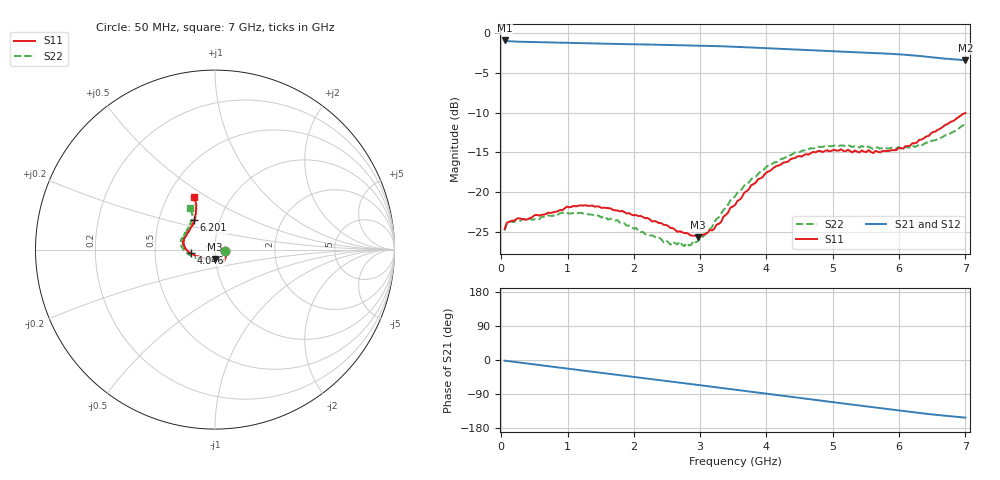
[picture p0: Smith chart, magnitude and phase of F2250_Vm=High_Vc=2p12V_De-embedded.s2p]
! Integrated Device Technology
! Corporate Headquarters
! 6024 Silver Creek Valley Road
! San Jose, CA 95138  USA
! Phone:  1-408-284-8200
! Toll Free:  1-800-223-1366
! Webpage:  http://www.idt.com/
! Timing and RF Division
! 515 Groton Road, Suite 102
! Westford, MA 01886-6024
! Device:  F2250
! Description: Voltage Variable RF Attenuator
! Frequency:  50.0 -  6000.00 MHz
! Package:  3x3 mm Thin QFN Plastic Package: 16 pin
! Ports:  2 RF, 3 DC
!  Pin  1  = GND
!  Pin  2  = NC
!  Pin  3  = RF1  = Port 1
!  Pin  4  = NC
!  Pin  5  = GND
!  Pin  6  = GND
!  Pin  7  = GND
!  Pin  8  = GND
!  Pin  9  = NC
!  Pin 10  = RF2  = Port 2
!  Pin 11  = NC
!  Pin 12  = GND
!  Pin 13  = GND
!  Pin 14  = VCNTRL
!  Pin 15  = VDD
!  Pin 16  = VMODE
! Vcntrl:  2.120 Volts
! Vmode:  +3.300 Volts
! Vdd:  +3.30  Volts
! Current:  1.316 mA
! Data:  The device was measured on a the F2250 evaluation board which has
!  individual transmission lines to the RF pins.  Data was collected
!  using a calibrated network analyzer.  The evaluation board was
!  de-embedded using a TRL calibration technique.
!  The reference plane is the edge of the package pin.
! Misc:  SN 10
!  Action Tracker AT0258
! Date Measured:  2014-11-26
! Date:  2015-10-15  MJV
! Note:
!  Integrated Device Technology supplies this data as a sample of measured
!  data at the package pin for this product.  Your particular data for this
!  product may vary.
!  Data was taken at 25 degrees C.
!  Integrated Device Technology reserves the right to change this data at anytime.
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# GHz S dB R 50
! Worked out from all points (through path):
!   201 points, 50 MHz to 7 GHz, reference 50 ohm
!   highest |S21| = -0.96 dB at 50 MHz (marker M1); lowest = -3.4 dB at 7 GHz (marker M2)
!   group delay of S21, straight-line fit = 61.1 ps
!   lowest |S11| = -25.6 dB at 2.969 GHz (marker M3), VSWR 1.11, Z = 49.6 - j5.19 ohm
!   |S11| at or under -10 dB: start of sweep to end of sweep
!   |S22| runs from -26.8 to -11.5 dB; largest |S21 - S12| = 0.0019
!   S11 on the Smith chart (normalised r, x): 50 MHz: 1.12, -0.02; 4.046 GHz: 0.76, -0.03; 6.201 GHz: 0.75, +0.26; 7 GHz: 0.68, +0.44
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0.05  -24.60 -9.5  -0.96 -1.8  -0.95 -1.8  -24.80 -10.0
0.08475  -23.83 -8.6  -1.03 -2.5  -1.02 -2.5  -23.89 -8.9
0.1195  -23.72 -9.3  -1.06 -3.3  -1.05 -3.2  -23.71 -8.3
0.91875  -22.27 -46.8  -1.24 -21.0  -1.24 -21.1  -22.56 -49.1
1.2315  -21.69 -54.6  -1.31 -27.9  -1.31 -27.9  -22.67 -59.5
1.75275  -22.29 -61.5  -1.40 -39.1  -1.40 -39.1  -23.49 -66.7
2.37825  -23.88 -61.7  -1.49 -52.8  -1.50 -52.8  -25.70 -68.5
2.552  -24.48 -66.1  -1.52 -56.6  -1.52 -56.6  -26.58 -75.0
2.691  -24.90 -73.4  -1.54 -59.7  -1.54 -59.7  -26.19 -82.3
2.7605  -25.14 -75.3  -1.56 -61.3  -1.56 -61.3  -26.77 -86.6
2.969  -25.64 -91.7  -1.59 -66.0  -1.59 -66.0  -26.13 -104.5
3.21225  -24.58 -121.1  -1.65 -71.4  -1.65 -71.5  -23.73 -128.6
3.525  -21.62 -147.8  -1.75 -78.5  -1.75 -78.5  -20.52 -147.2
3.76825  -19.13 -161.2  -1.84 -84.0  -1.84 -84.0  -18.38 -158.4
4.04625  -17.35 -171.2  -1.95 -90.2  -1.95 -90.2  -16.70 -168.9
4.4285  -15.72 178.2  -2.10 -98.6  -2.10 -98.6  -15.01 179.5
4.7065  -14.94 171.1  -2.20 -104.8  -2.20 -104.8  -14.51 173.6
5.054  -14.79 162.9  -2.33 -112.4  -2.32 -112.5  -14.12 166.5
5.85325  -14.81 136.7  -2.62 -130.0  -2.62 -130.1  -14.53 147.6
6.20075  -13.85 124.9  -2.83 -137.7  -2.83 -137.8  -14.13 138.5
6.54825  -12.39 116.7  -3.10 -144.7  -3.11 -144.8  -13.48 127.1
7  -10.07 111.6  -3.43 -152.0  -3.44 -152.2  -11.48 120.8
